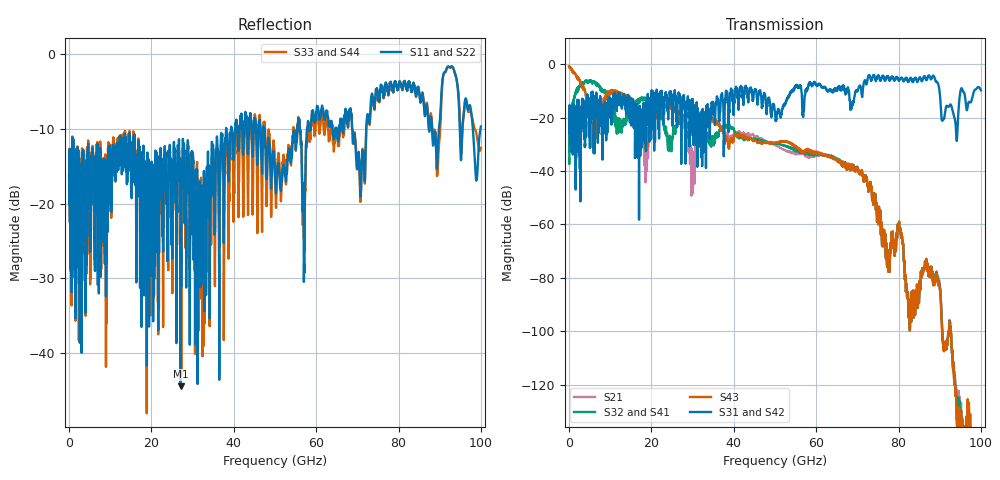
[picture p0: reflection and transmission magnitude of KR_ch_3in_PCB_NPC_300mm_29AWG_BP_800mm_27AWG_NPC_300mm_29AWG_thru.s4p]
# GHz S RI R 45
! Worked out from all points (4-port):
!   4000 points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, 25 MHz to 100 GHz, reference 45 ohm
!   strongest paths, dB at 25 MHz, 25.02 GHz, 50.02 GHz, 75.03 GHz, 100 GHz:
!     S31: -20.6, -18.1, -18.0, -4.3, -9.7
!     S42: -20.6, -18.0, -18.0, -4.3, -9.8
!     S43: -0.8, -15.7, -29.5, -57.7, -144.8
!     S32: -35.3, -28.8, -29.7, -57.8, -152.3
!     S41: -35.3, -28.8, -29.7, -57.8, -152.3
!     S21: -0.8, -15.7, -30.2, -57.9, -160.1
!   lowest |S11| = -44.4 dB at 27.1 GHz (marker M1), VSWR 1.01, Z = 44.9 - j0.529 ohm
!   |S11| at or under -10 dB: start of sweep to 38.14 GHz; 47.46 GHz to 55.41 GHz (7.945 GHz wide, 15.4 % of centre); 68.73 GHz to 72.16 GHz (3.431 GHz wide, 4.87 % of centre)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
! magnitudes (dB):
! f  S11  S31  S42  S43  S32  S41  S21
! 25 MHz  -16.1  -20.6  -20.6  -0.8  -35.3  -35.3  -0.8
! 4.125 GHz  -15.5  -16.8  -16.9  -11.8  -6.4  -6.4  -11.6
! 18.73 GHz  -17.3  -22.0  -22.1  -26.3  -13.3  -13.3  -30.0
! 27.1 GHz  -44.4  -17.5  -17.6  -18.5  -20.1  -20.1  -19.2
! 69.83 GHz  -14.9  -10.0  -10.2  -39.4  -39.3  -39.3  -39.1
! 77.4 GHz  -4.7  -4.7  -4.7  -72.2  -72.3  -72.3  -72.3
! 100 GHz  -9.7  -9.7  -9.8  -144.8  -152.3  -152.3  -160.1
